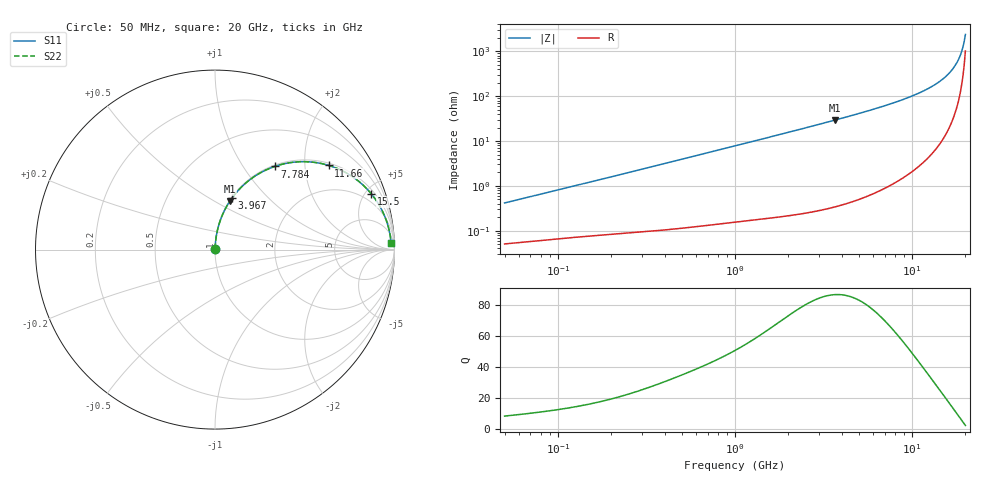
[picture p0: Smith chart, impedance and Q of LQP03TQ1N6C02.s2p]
!Murata Part Number: LQP03TQ1N6C02
!These Parameters are Measured in Series Mode Connection
!  o--[Z]--o
!Port1  Port2
!  o-------o
!Freq. Start=50[MHz] Stop=20[GHz], 401[Steps]
# Hz S RI R 50
!Freq.(Hz) S11(Real) S11(Imag) S21(Real) S21(Imag) S12(Real) S12(Imag) S22(Real) S22(Imag)
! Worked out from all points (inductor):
!   401 points, 50 MHz to 20 GHz, reference 50 ohm
!   read as one part in series: L = 1.3 nH near 51.52 MHz
!   highest Q = 86.5 at 3.681 GHz (marker M1), where L = 1.27 nH
!   S11 on the Smith chart (normalised r, x): 50 MHz: 1.00, +0.01; 3.967 GHz: 1.01, +0.64; 7.784 GHz: 1.02, +1.40; 11.66 GHz: 1.07, +2.65; 15.5 GHz: 1.28, +5.50; 20 GHz: 21, +43
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5e7  0.000522 0.00411  0.9995 -0.00411  0.9995 -0.00411  0.000522 0.00411
1.364002e8  0.00085 0.0109  0.9992 -0.0109  0.9992 -0.0109  0.00085 0.0109
3.721004e8  0.00186 0.0291  0.9981 -0.0291  0.9981 -0.0291  0.00186 0.0291
1e9  0.00755 0.0772  0.9924 -0.0772  0.9924 -0.0772  0.00755 0.0772
1.714689e9  0.0195 0.1309  0.9805 -0.1309  0.9805 -0.1309  0.0195 0.1309
2.728004e9  0.0464 0.2043  0.9536 -0.2043  0.9536 -0.2043  0.0464 0.2043
3.680849e9  0.0821 0.2688  0.9179 -0.2688  0.9179 -0.2688  0.0821 0.2688
3.967106e9  0.0948 0.2872  0.9052 -0.2872  0.9052 -0.2872  0.0948 0.2872
5.598765e9  0.1821 0.3797  0.8179 -0.3797  0.8179 -0.3797  0.1821 0.3797
7.442007e9  0.3068 0.4537  0.6932 -0.4537  0.6932 -0.4537  0.3068 0.4537
7.784049e9  0.3321 0.4632  0.6679 -0.4632  0.6679 -0.4632  0.3321 0.4632
9.745021e9  0.4847 0.4899  0.5153 -0.4899  0.5153 -0.4899  0.4847 0.4899
1.166392e10  0.6338 0.469  0.3662 -0.469  0.3662 -0.469  0.6338 0.469
1.375312e10  0.7773 0.3984  0.2227 -0.3984  0.2227 -0.3984  0.7773 0.3984
1.550395e10  0.8714 0.3102  0.1286 -0.3102  0.1286 -0.3102  0.8714 0.3102
1.696185e10  0.9277 0.2245  0.0723 -0.2245  0.0723 -0.2245  0.9277 0.2245
1.800918e10  0.9555 0.1596  0.0445 -0.1596  0.0445 -0.1596  0.9555 0.1596
1.855685e10  0.9659 0.1254  0.0341 -0.1254  0.0341 -0.1254  0.9659 0.1254
1.88369e10  0.9702 0.108  0.0298 -0.108  0.0298 -0.108  0.9702 0.108
1.912117e10  0.9739 0.0903  0.0261 -0.0903  0.0261 -0.0903  0.9739 0.0903
1.970266e10  0.9792 0.0545  0.0208 -0.0545  0.0208 -0.0545  0.9792 0.0545
2e10  0.981 0.0365  0.019 -0.0365  0.019 -0.0365  0.981 0.0365
